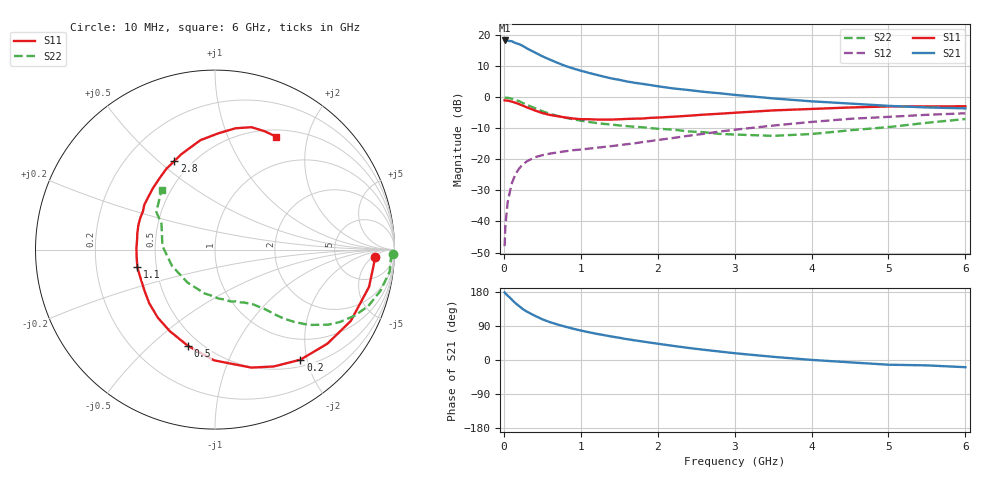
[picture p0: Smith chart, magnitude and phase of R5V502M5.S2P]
! SIEMENS Small Signal Semiconductors
! BFR183
! Si NPN RF Bipolar Junction Transistor in SOT23
! VCE = 0.5 V  IC = 2.5 mA
! Common Emitter S-Parameters:  May  1996
# GHz  S  MA  R  50
!  f  S11  S21  S12  S22
! GHz  MAG  ANG  MAG  ANG  MAG  ANG  MAG  ANG
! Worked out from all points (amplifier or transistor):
!   36 points, 10 MHz to 6 GHz, reference 50 ohm
!   highest |S21| = 18.3 dB at 10 MHz (marker M1)
!   |S21| within 3 dB of that: start of sweep to 335 MHz
!   unconditionally stable (mu >= 1): 1.219 GHz to 3.52 GHz
!   at 250 MHz: K = 0.28, MSG = 19.0 dB, |S12| = -21.6 dB
!   at 1.4 GHz: K = 1.08, MAG = 9.2 dB, |S12| = -15.7 dB
!   at 6 GHz: K = 0.99, MSG = 0.8 dB, |S12| = -5.2 dB
!   S11 on the Smith chart (normalised r, x): 10 MHz: 15, -6; 200 MHz: 0.61, -1.88; 500 MHz: 0.43, -0.67; 1.1 GHz: 0.39, -0.10; 2.8 GHz: 0.40, +0.57; 6 GHz: 0.59, +1.51
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0.01  0.8926 -2.8  8.231 178.4  0.004 89.8  0.9917 -1.4
0.02  0.8881 -5.6  8.095 175.8  0.0085 88.7  0.9811 -2.9
0.05  0.883 -13.6  8.118 169.9  0.0205 81.9  0.9808 -7.2
0.1  0.8547 -27.7  8.014 160.1  0.0399 75.4  0.95 -14.0
0.15  0.8166 -39.9  7.493 150.3  0.0574 68.0  0.9102 -20.2
0.2  0.7764 -52.2  7.166 141.9  0.0717 62.2  0.8613 -25.3
0.25  0.7288 -63.3  6.681 134.0  0.0834 57.0  0.8044 -30.1
0.3  0.6878 -72.9  6.133 127.6  0.0931 53.4  0.756 -33.6
0.4  0.617 -90.5  5.299 117.1  0.1077 47.3  0.6714 -38.7
0.5  0.5573 -105.6  4.579 107.4  0.1169 43.3  0.5975 -42.4
0.6  0.5196 -119.0  4.034 99.9  0.124 40.8  0.5417 -45.1
0.7  0.4952 -130.1  3.582 93.5  0.1297 39.2  0.5006 -46.9
0.9  0.4548 -149.7  2.916 82.6  0.1406 37.8  0.4428 -49.5
1.1  0.4438 -167.1  2.483 73.5  0.1488 38.2  0.4024 -52.4
1.4  0.4375 173.0  2.011 62.0  0.1634 39.5  0.3633 -56.7
1.6  0.4484 162.1  1.799 55.0  0.1754 40.5  0.3435 -59.9
2.2  0.486 135.6  1.39 37.3  0.2211 42.2  0.3019 -73.2
2.8  0.543 114.6  1.162 22.5  0.2799 40.4  0.2575 -94.2
3.5  0.6151 97.6  0.96 8.4  0.3503 33.9  0.2391 -130.0
4.5  0.6856 80.4  0.793 -6.2  0.4501 21.5  0.2939 175.9
5.5  0.715 67.2  0.686 -14.2  0.5227 9.2  0.3884 147.3
6  0.7157 61.6  0.663 -19.0  0.5523 1.2  0.4469 131.7
